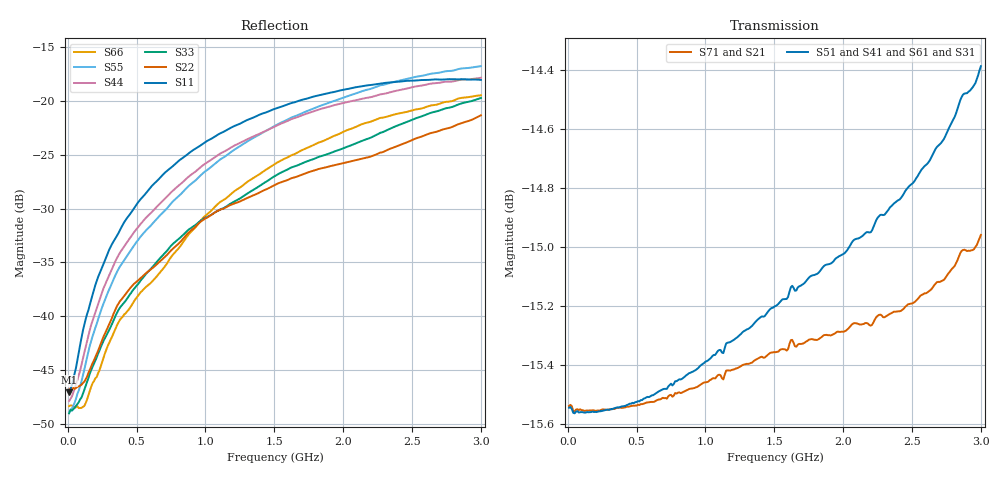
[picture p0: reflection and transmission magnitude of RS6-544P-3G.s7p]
! MTS Systemtechnik GmbH
! S-Parameters
! Model: z.B.: RS6-544P-3G
! Rohde & Schwarz ZVB8 2Ports - Version 3.20 - 1145.1010k08 SN: 100119
! Converted & adapted with MATLAB
!  OUT 2 (Port 3)
!  o
! OUT 1 (Port 2) o  /  MTS  \  o OUT 3 (Port 4)
!  C (Port 1) o--|  RS6-544P-3G  |
! OUT 6 (Port 7) o  \  /  o OUT 4 (Port 5)
!  o
!  OUT 5 (Port 6)
! S7P File: Measurements:
! <S11,S12,S13,S14,S15,S16,S17>,
! <S21,S22,S23,S24,S25,S26,S27>,
! <S31,S32,S33,S34,S35,S36,S37>,
! <S41,S42,S43,S44,S45,S46,S47>,
! <S51,S52,S53,S54,S55,S56,S57>,
! <S61,S62,S63,S64,S65,S66,S67>,
! <S71,S72,S73,S74,S75,S76,S77>:
# HZ  S  DB  R  50.00
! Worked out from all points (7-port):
!   300 points, 10 MHz to 3 GHz, reference 50 ohm
!   strongest paths, dB at 10 MHz, 760 MHz, 1.51 GHz, 2.26 GHz, 3 GHz:
!     S51: -15.5, -15.5, -15.2, -14.9, -14.4
!     S41: -15.5, -15.5, -15.2, -14.9, -14.4
!     S61: -15.5, -15.5, -15.2, -15.0, -14.5
!     S31: -15.5, -15.5, -15.3, -15.0, -14.6
!     S71: -15.5, -15.5, -15.4, -15.2, -15.0
!     S21: -15.5, -15.5, -15.4, -15.3, -15.0
!   lowest |S11| = -47.1 dB at 10 MHz (marker M1), VSWR 1.01, Z = 49.6 - j0.0607 ohm
!   |S11| at or under -10 dB: start of sweep to end of sweep
